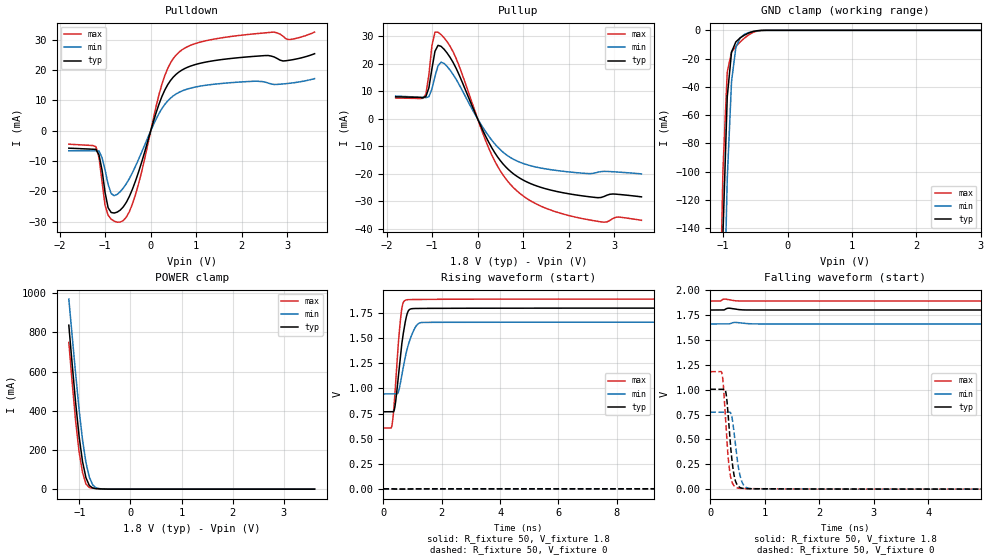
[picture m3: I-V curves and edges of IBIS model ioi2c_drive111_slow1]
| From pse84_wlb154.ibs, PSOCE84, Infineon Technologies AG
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[Model] ioi2c_drive111_slow1
Model_type I/O
Enable   Active-High
Vinl  =  0.54
Vinh  =  1.26
Vmeas =  0.9
Cref  =  15e-12
| Capacitance   typ   min   max
C_comp   8.55364e-13 8.30808e-13 8.84570e-13
| Variables   typ   min   max
[GND Clamp Reference]   0   0   0
[POWER Clamp Reference]   1.8   1.66   1.89
[Pulldown Reference]   0   0   0
[Pullup Reference]   1.8   1.66   1.89
[Temperature Range]   25   125   -40
[Voltage Range]   1.8   1.66   1.89
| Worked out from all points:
|   slope of the pulldown table from 0 to 0.27 V, typ, clamps not added: 22.3 ohm
|   slope of the pullup table from 0 to 0.27 V, typ, clamps not added: 29.1 ohm
|   GND clamp passes 1 mA (typ) near -0.55 V on its own axis
|   POWER clamp passes 1 mA (typ) near -0.55 V on its own axis
|   falling waveform, R_fixture 50, V_fixture 1.8: 20-80 % time 99.8ns typ, 151ns min, 56.6ns max; typ from 1.8 V to 0.767 V
|   falling waveform, R_fixture 50, V_fixture 0: 20-80 % time 98.8ps typ, 113ps min, 90.7ps max; typ from 1 V to 0 V
|   rising waveform, R_fixture 50, V_fixture 1.8: 20-80 % time 247ps typ, 344ps min, 193ps max; typ from 0.767 V to 1.8 V
|   rising waveform, R_fixture 50, V_fixture 0: 20-80 % time 104ns typ, 159ns min, 61.6ns max; typ from 0 V to 1 V
[GND Clamp]
| Voltage   I(typ)   I(min)   I(max)
-1.204V   -750.5mA   -844.3mA   -692.2mA
-1.07V    -311.8mA   -416.8mA   -250.3mA
-1.003V   -144.6mA   -236.7mA   -99.35mA
-936.6mV  -47.15mA   -105.3mA   -29.57mA
-869.7mV  -15.32mA   -36.11mA   -15.4mA
-802.8mV  -8.178mA   -12.13mA   -11.32mA
-735.9mV  -5.345mA   -5.294mA   -8.218mA
-669mV    -3.361mA   -2.852mA   -5.471mA
-535.2mV  -838.5uA   -772.4uA   -1.486mA
-401.4mV  -47.36uA   -84.85uA   -76.78uA
3.6V      0A         0A         0A
[POWER Clamp]
| Voltage   I(typ)   I(min)   I(max)
-1.204V   837.3mA    970.7mA    749.2mA
-1.137V   634.9mA    778.2mA    540.5mA
-1.07V    440.1mA    587.4mA    346.5mA
-1.003V   270mA      407mA      190.9mA
-936.6mV  141.8mA    252.7mA    85.92mA
-869.7mV  58.74mA    136.5mA    26.66mA
-802.8mV  18.35mA    60.36mA    8.197mA
-735.9mV  5.885mA    21mA       4.755mA
-669mV    2.866mA    6.628mA    3.138mA
-334.5mV  12.31uA    45.7uA     5.857uA
3.6V      0A         0A         0A
[Pulldown]
| Voltage   I(typ)   I(min)   I(max)
-1.8V     -5.733mA   -6.581mA   -4.412mA
-1.204V   -6.135mA   -6.635mA   -5.251mA
-1.07V    -12.91mA   -8.838mA   -16.71mA
-1.003V   -20.34mA   -12.88mA   -24.59mA
-936.6mV  -25.37mA   -17.69mA   -27.83mA
-802.8mV  -27.11mA   -21.39mA   -29.79mA
-669mV    -26.13mA   -20.05mA   -30.08mA
-334.5mV  -16.53mA   -11.66mA   -21.01mA
310.3mV   13.46mA    8.709mA    18.26mA
620.7mV   19.37mA    12.66mA    25.9mA
1.614V    23.57mA    15.67mA    30.76mA
3.6V      25.4mA     17.19mA    32.52mA
[Pullup]
| Voltage   I(typ)   I(min)   I(max)
-1.8V     7.982mA    8.271mA    7.548mA
-1.137V   8.074mA    7.699mA    8.897mA
-1.07V    11.27mA    8.018mA    16.05mA
-1.003V   18.24mA    10.84mA    26.64mA
-936.6mV  24.54mA    15.47mA    31.51mA
-869.7mV  26.7mA     19.31mA    31.46mA
-735.9mV  25.25mA    20.1mA     29.42mA
-468.3mV  18.22mA    14.25mA    21.81mA
372.4mV   -12.19mA   -9mA       -15.2mA
869mV     -20.94mA   -15.34mA   -26.26mA
2.126V    -27.56mA   -19.48mA   -35.61mA
3.6V      -28.34mA   -20mA      -36.86mA
[Ramp]
dV/dt_r   0.602353/0.104189u  0.463505/0.159188u  0.708541/61.6075n
dV/dt_f   0.619713/99.7907n  0.428618/0.150856u  0.770746/56.6345n
R_load = 50
[Falling Waveform]
R_fixture = 50
V_fixture = 1.8
V_fixture_min = 1.66
V_fixture_max = 1.89
| Time   V(typ)   V(min)   V(max)
0s        1.8V       1.66V      1.89V
10.41ns   1.8V       1.66V      1.865V
20.09ns   1.769V     1.658V     1.673V
37.51ns   1.607V     1.618V     1.332V
62.58ns   1.376V     1.511V     996.8mV
87.66ns   1.197V     1.403V     806.5mV
129.5ns   1.003V     1.257V     671.9mV
204.9ns   846.1mV    1.098V     615.7mV
321.6ns   782.2mV    996.1mV    606.1mV
800ns     767.1mV    945.6mV    605.4mV
[Falling Waveform]
R_fixture = 50
V_fixture = 0
V_fixture_min = 0
V_fixture_max = 0
| Time   V(typ)   V(min)   V(max)
0s        1.004V     773.6mV    1.181V
216.8ps   1.004V     773.6mV    1.157V
243.6ps   1.004V     773.6mV    1.017V
294.9ps   940.7mV    773.5mV    561.4mV
355.3ps   542.3mV    773.9mV    180.4mV
423.9ps   179.2mV    623.4mV    41.71mV
523.5ps   24.69mV    194.7mV    9.019mV
627.5ps   6.472mV    29.49mV    6.081mV
1.651ns   1.861mV    1.58mV     1.73mV
800ns     6.286nV    434.1nV    2.309nV
[Rising Waveform]
R_fixture = 50
V_fixture = 1.8
V_fixture_min = 1.66
V_fixture_max = 1.89
| Time   V(typ)   V(min)   V(max)
0s        767.1mV    945mV      605.4mV
302.4ps   767.2mV    945mV      646.9mV
406.3ps   839.8mV    945.1mV    995mV
495ps     1.073V     952.8mV    1.383V
565.7ps   1.28V      1.028V     1.63V
678.9ps   1.542V     1.206V     1.854V
850.5ps   1.771V     1.431V     1.884V
1.158ns   1.796V     1.636V     1.886V
2.065ns   1.798V     1.659V     1.888V
800ns     1.8V       1.66V      1.89V
[Rising Waveform]
R_fixture = 50
V_fixture = 0
V_fixture_min = 0
V_fixture_max = 0
| Time   V(typ)   V(min)   V(max)
0s        6.219nV    430.9nV    2.302nV
12.92ns   301.7uV    -64.05uV   23.28mV
24.26ns   42.53mV    5.727mV    207.1mV
49.64ns   262.1mV    88.66mV    607.7mV
77.63ns   482.7mV    214.9mV    883.1mV
102.7ns   632.7mV    318.4mV    1.016V
144.5ns   796.4mV    457mV      1.115V
218.5ns   928.1mV    610.9mV    1.166V
341.4ns   988.1mV    719.2mV    1.179V
800ns     1.004V     772.5mV    1.181V
